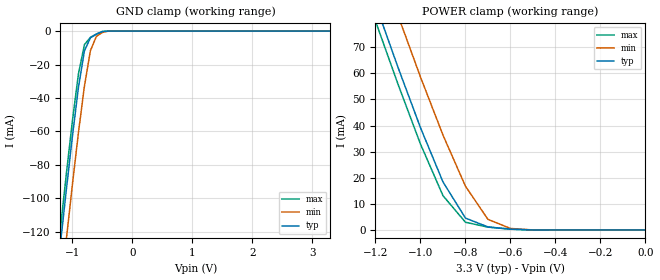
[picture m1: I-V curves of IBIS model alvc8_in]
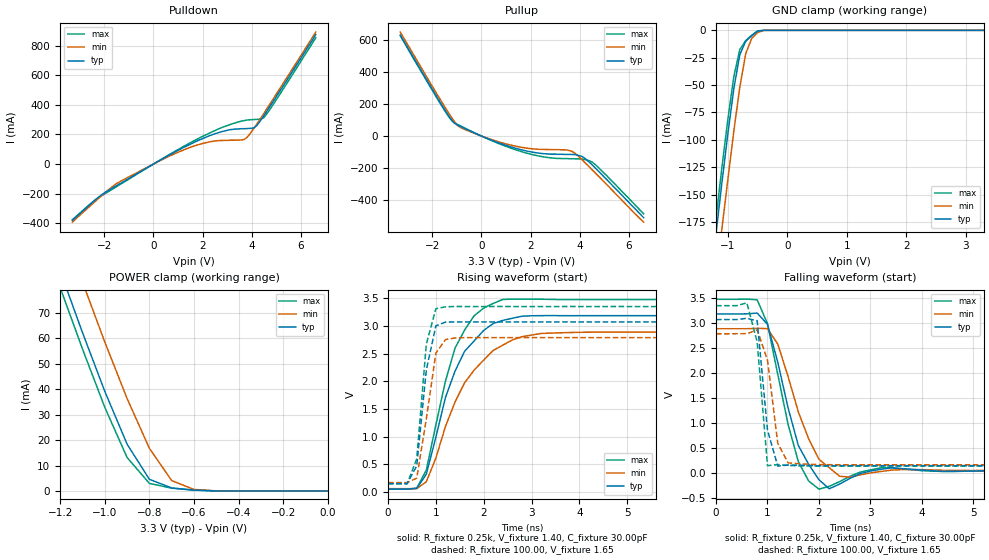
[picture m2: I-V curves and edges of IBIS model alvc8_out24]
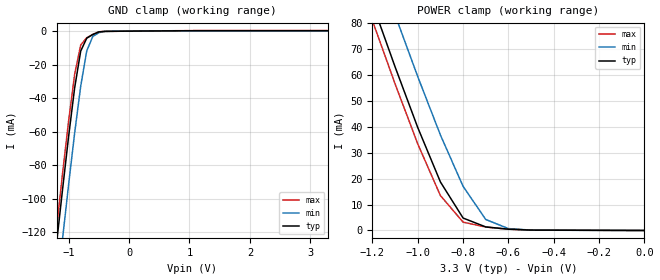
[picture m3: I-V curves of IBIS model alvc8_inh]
| IBIS file 16244ah.ibs created by s2ibis2 version 1.1
| North Carolina State University Electronics Research Laboratory  1995
[IBIS ver]   2.1
[File name]   16244ah.ibs
[File Rev]   1.0
[Date]   03/01/99 rtk rtk
[Source]   Integrated Device Technology, Inc.
[Notes]   1.Temperatures: typ=25C, min=100C, max=0C 2.RRmp rates based
   on 50 ohm load.
[Disclaimer] Integrated Device Technology, Inc. ("IDT") hereby grants the
   user of this IBIS model a non-exclusive, nontransferable
   license to use this IBIS model under the following terms. The
   user is granted this license only to use the IBIS model and is
   not granted rights to sell, copy (except as needed to run the
   IBIS model), rent, lease or sub-license the IBIS model in
   whole or in part, or in modified form to anyone. The User may
   modify the IBIS model to suit its specific applications, but
   rights to derivative works and such modifications shall belong
   to IDT. This IBIS model is provided on an AS IS" basis and IDT
   makes absolutely no warranty with respect to the information
   contained herein. IDT DISCLAIMS AND CUSTOMER WAIVES ALL
   WARRANTIES, EXPRESS AND IMPLIED, INCLUDING WARRANTIES OF
   MERCHANTABILITY AND FITNESS FOR A PARTICULAR PURPOSE. THE
   ENTIRE RISK AS TO QUALITY AND PERFORMANCE IS WITH THE USER
   ACCORDINGLY, IN NO EVENT SHALL IDT BE LIABLE FOR ANY DIRECT OR
   INDIRECT DAMAGES, WHETHER IN CONTRACT OR TORT, INCLUDING ANY
   LOST PROFITS OR OTHER INCIDENTAL, CONSEQUENTIAL, EXEMPLARY, OR
   PUNITIVE DAMAGES ARISING OUT OF THE USE OR APPLICATION OF THE
   IBIS model. Further, IDT reserves the right to make changes
   without notice to any product herein to improve reliability,
   function, or design. IDT does not convey any license under
   patent rights or any other intellectual property rights,
   including those of third parties. IDT is not obligated to
   provide maintenance or support for the licensed IBIS model.
[Copyright]   Copyright 1997, Integrated Device Technology, Inc. all rights
   reserved
|   Component ALVCH16244
[Component]   ALVCH16244
[Manufacturer]   Integrated Device Technology
[Package]
| PA48
| variable   typ   min   max
R_pkg   6.50m   5.00m   10.00m
L_pkg   3.20nH   2.50nH   4.40nH
C_pkg   0.27pF   0.01pF   0.98pF
| PV48   typ   min   max
|R_pkg   6.5m   5.00m   10.00m
|L_pkg   4.75nH   3.82nH   6.72nH
|C_pkg   0.24pF   0.01pF   1.55pF
[Pin]  signal_name   model_name   R_pin   L_pin   C_pin
1   1OEB   alvc8_in
2   1Y1   alvc8_out24
3   1Y2   alvc8_out24
4   GND   GND
5   1Y3   alvc8_out24
6   1Y4   alvc8_out24
7   VCC   POWER
8   2Y1   alvc8_out24
9   2Y2   alvc8_out24
10   GND   GND
11   2Y3   alvc8_out24
12   2Y4   alvc8_out24
13   3Y1   alvc8_out24
14   3Y2   alvc8_out24
15   GND   GND
16   3Y3   alvc8_out24
17   3Y4   alvc8_out24
18   VCC   POWER
19   4Y1   alvc8_out24
20   4Y2   alvc8_out24
21   GND   GND
22   4Y3   alvc8_out24
23   4Y4   alvc8_out24
24   4OEB   alvc8_in
25   3OEB   alvc8_in
26   4A4   alvc8_inh
27   4A3   alvc8_inh
28   GND   GND
29   4A2   alvc8_inh
30   4A1   alvc8_inh
31   VCC   POWER
32   3A4   alvc8_inh
33   3A3   alvc8_inh
34   GND   GND
35   3A2   alvc8_inh
36   3A1   alvc8_inh
37   2A4   alvc8_inh
38   2A3   alvc8_inh
39   GND   GND
40   2A2   alvc8_inh
41   2A1   alvc8_inh
42   VCC   POWER
43   1A4   alvc8_inh
44   1A3   alvc8_inh
45   GND   GND
46   1A2   alvc8_inh
47   1A1   alvc8_inh
48   2OEB   alvc8_in
| Models and submodels in the file (3): alvc8_in (Input), alvc8_out24 (3-state), alvc8_inh (Input)
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| in   in   dummy_model
| oe   oe   dummy_model
|   Model alvc8_in
[Model]   alvc8_in
Model_type   Input
Vinl =  0.800V
Vinh =  2.000V
C_comp   3.00pF   NA   NA
[Temperature Range]   25.00   100.00   0.000
[Voltage Range]   3.30V   3.00V   3.60V
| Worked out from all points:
|   GND clamp passes 1 mA (typ) near -0.54 V on its own axis
|   POWER clamp passes 1 mA (typ) near -0.68 V on its own axis
[GND_clamp]
| voltage   I(typ)   I(min)   I(max)
-3.3V     -860mA     -887mA     -851mA
-1.3V     -161mA     -190mA     -151mA
-1.2V     -127mA     -157mA     -118mA
-1.1V     -94.41mA   -124mA     -84.85mA
-1V       -62.78mA   -91.54mA   -53.52mA
-900mV    -33.71mA   -60.78mA   -25.6mA
-800mV    -11.74mA   -32.83mA   -8.09mA
-700mV    -4.033mA   -11.65mA   -3.7mA
-600mV    -1.899mA   -3.108mA   -1.699mA
-500mV    -308uA     -810uA     -172uA
-400mV    -3.848nA   -9.872uA   -399pA
3.3V      39.6pA     19.33nA    26.4pA
[POWER_clamp]
| voltage   I(typ)   I(min)   I(max)
-3.3V     630mA      648mA      624mA
-1.2V     86.56mA    106mA      80.02mA
-1.1V     62.33mA    82.22mA    55.88mA
-1V       39.2mA     58.61mA    32.91mA
-900mV    18.4mA     36.35mA    13.15mA
-800mV    4.556mA    16.76mA    2.954mA
-700mV    1.164mA    4.056mA    1.087mA
-600mV    320uA      578uA      299uA
-500mV    40.08nA    12.23uA    3.465nA
0V        39.6pA     59.11pA    43.2pA
|   Model alvc8_out24
[Model]   alvc8_out24
Model_type   3-state
Polarity   Non-Inverting
Enable   Active-High
Vmeas =  1.500V
C_comp   3.00pF   NA   NA
[Temperature Range]   25.00   100.00   0.000
[Voltage Range]   3.30V   3.00V   3.60V
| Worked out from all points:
|   slope of the pulldown table from 0 to 0.495 V, typ, clamps not added: 10.5 ohm
|   slope of the pullup table from 0 to 0.495 V, typ, clamps not added: 16.1 ohm
|   GND clamp passes 1 mA (typ) near -0.50 V on its own axis
|   POWER clamp passes 1 mA (typ) near -0.68 V on its own axis
|   rising waveform, R_fixture 0.25k, V_fixture 1.40, C_fixture 30.00pF: 20-80 % time 712ps typ, 930ps min, 636ps max; typ from 0.056 V to 3.19 V
|   rising waveform, R_fixture 100.00, V_fixture 1.65: 20-80 % time 241ps typ, 276ps min, 194ps max; typ from 0.155 V to 3.08 V
|   falling waveform, R_fixture 0.25k, V_fixture 1.40, C_fixture 30.00pF: 20-80 % time 456ps typ, 551ps min, 426ps max; typ from 3.19 V to 0.056 V
|   falling waveform, R_fixture 100.00, V_fixture 1.65: 20-80 % time 185ps typ, 189ps min, 171ps max; typ from 3.08 V to 0.155 V
[Pulldown]
| voltage   I(typ)   I(min)   I(max)
-3.3V     -381mA     -393mA     -377mA
-2.2V     -219mA     -227mA     -224mA
-1.5V     -146mA     -132mA     -153mA
500mV     47.5mA     41.7mA     49.9mA
1.4V      126mA      107mA      135mA
2.3V      193mA      151mA      211mA
3.1V      232mA      161mA      266mA
3.7V      239mA      167mA      294mA
4.1V      246mA      246mA      301mA
4.5V      329mA      345mA      316mA
5.1V      483mA      500mA      461mA
6.6V      875mA      892mA      853mA
[Pullup]
| voltage   I(typ)   I(min)   I(max)
-3.3V     630mA      649mA      628mA
-1.4V     142mA      160mA      137mA
-1.1V     80.6mA     90.7mA     83.6mA
-900mV    63mA       57.7mA     67.6mA
400mV     -25.1mA    -21.5mA    -27.4mA
1.6V      -85mA      -69.5mA    -95.9mA
2.6V      -111mA     -84mA      -132mA
3.4V      -115mA     -86.1mA    -141mA
3.7V      -115mA     -97.1mA    -142mA
4.1V      -128mA     -149mA     -144mA
4.5V      -179mA     -210mA     -162mA
6.6V      -510mA     -538mA     -486mA
[GND_clamp]
| voltage   I(typ)   I(min)   I(max)
-3.3V     -1.227A    -1.266A    -1.214A
-1.3V     -233mA     -276mA     -219mA
-1.2V     -186mA     -228mA     -172mA
-1.1V     -139mA     -181mA     -125mA
-1V       -94.27mA   -136mA     -81.1mA
-900mV    -53.23mA   -91.93mA   -42.09mA
-800mV    -22.31mA   -52.04mA   -17.61mA
-700mV    -9.958mA   -21.29mA   -9.325mA
-600mV    -4.943mA   -7.436mA   -4.424mA
-500mV    -830uA     -2.115mA   -472uA
-400mV    -8.73nA    -25.66uA   -695pA
3.3V      92.41pA    19.42nA    79.2pA
[POWER_clamp]
| voltage   I(typ)   I(min)   I(max)
-3.3V     630mA      648mA      624mA
-1.2V     86.56mA    106mA      80.02mA
-1.1V     62.33mA    82.22mA    55.88mA
-1V       39.2mA     58.61mA    32.91mA
-900mV    18.4mA     36.35mA    13.15mA
-800mV    4.556mA    16.76mA    2.954mA
-700mV    1.164mA    4.056mA    1.087mA
-600mV    320uA      578uA      299uA
-500mV    40.14nA    12.23uA    3.53nA
0V        92.41pA    138pA      101pA
[Ramp]
| variable   typ   min   max
dV/dt_r   1.48/0.31n   1.29/0.30n   1.66/0.22n
dV/dt_f   1.63/0.28n   1.45/0.31n   1.80/0.19n
R_load = 50.00
[Rising Waveform]
R_fixture = 0.25k
V_fixture = 1.40
C_fixture = 30.00pF
R_dut = 7.00m
L_dut = 3.30nH
C_dut = 0.29pF
| time   V(typ)   V(min)   V(max)
0s        55.61mV    62.15mV    53.22mV
600ps     67.1mV     63.76mV    71.36mV
800ps     323mV      188mV      399mV
1.2ns     1.71V      1.187V     2.006V
1.4ns     2.186V     1.627V     2.602V
1.8ns     2.733V     2.205V     3.187V
2.4ns     3.104V     2.656V     3.482V
2.8ns     3.179V     2.809V     3.489V
4ns       3.189V     2.888V     3.48V
19.8ns    3.189V     2.893V     3.481V
[Rising Waveform]
R_fixture = 100.00
V_fixture = 1.65
R_dut = 7.00m
L_dut = 3.30nH
C_dut = 0.29pF
| time   V(typ)   V(min)   V(max)
0s        155mV      173mV      149mV
400ps     155mV      173mV      149mV
600ps     476mV      252mV      604mV
800ps     2.207V     1.324V     2.674V
1ns       3.005V     2.511V     3.315V
1.2ns     3.072V     2.757V     3.349V
1.4ns     3.076V     2.786V     3.355V
1.6ns     3.076V     2.793V     3.354V
19.8ns    3.076V     2.792V     3.354V
[Falling Waveform]
R_fixture = 0.25k
V_fixture = 1.40
C_fixture = 30.00pF
R_dut = 7.00m
L_dut = 3.30nH
C_dut = 0.29pF
| time   V(typ)   V(min)   V(max)
0s        3.189V     2.893V     3.481V
800ps     3.206V     2.901V     3.471V
1ns       2.981V     2.895V     2.993V
1.2ns     2.223V     2.586V     1.98V
1.6ns     557mV      1.227V     234mV
2ns       -126mV     283mV      -314mV
2.2ns     -306mV     114mV      -257mV
2.4ns     -213mV     -54.48mV   -163mV
3.2ns     82.67mV    38.85mV    114mV
19.8ns    55.61mV    62.15mV    53.23mV
[Falling Waveform]
R_fixture = 100.00
V_fixture = 1.65
R_dut = 7.00m
L_dut = 3.30nH
C_dut = 0.29pF
| time   V(typ)   V(min)   V(max)
0s        3.076V     2.792V     3.354V
400ps     3.076V     2.793V     3.354V
600ps     3.101V     2.794V     3.411V
800ps     3.052V     2.869V     2.626V
1ns       869mV      2.268V     155mV
1.2ns     147mV      602mV      178mV
1.4ns     168mV      211mV      161mV
2ns       153mV      177mV      149mV
2.8ns     155mV      173mV      149mV
19.8ns    155mV      173mV      149mV
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|   Model alvc8_inh
[Model]   alvc8_inh
Model_type   Input
Vinl =  0.800V
Vinh =  2.000V
C_comp   3.00pF   NA   NA
[Temperature Range]   25.00   100.00   0.000
[Voltage Range]   3.30V   3.00V   3.60V
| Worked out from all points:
|   GND clamp passes 1 mA (typ) near -0.53 V on its own axis
|   POWER clamp passes 1 mA (typ) near -0.66 V on its own axis
[GND_clamp]
| voltage   I(typ)   I(min)   I(max)
-3.3V     -860mA     -888mA     -852mA
-1.3V     -161mA     -190mA     -151mA
-1.2V     -127mA     -157mA     -118mA
-1.1V     -94.51mA   -124mA     -84.99mA
-1V       -62.91mA   -91.62mA   -53.71mA
-900mV    -33.88mA   -60.87mA   -25.82mA
-800mV    -11.92mA   -32.93mA   -8.306mA
-700mV    -4.211mA   -11.77mA   -3.908mA
-600mV    -2.051mA   -3.213mA   -1.882mA
-500mV    -472uA     -914uA     -379uA
-400mV    -144uA     -112uA     -169uA
3.3V      264uA      163uA      349uA
[POWER_clamp]
| voltage   I(typ)   I(min)   I(max)
-3.3V     638mA      656mA      632mA
-1.2V     87.67mA    108mA      81.05mA
-1.1V     63.19mA    83.28mA    56.62mA
-1V       39.75mA    59.43mA    33.41mA
-900mV    18.73mA    36.86mA    13.47mA
-800mV    4.8mA      17.05mA    3.222mA
-700mV    1.374mA    4.243mA    1.32mA
-600mV    498uA      728uA      497uA
-500mV    146uA      134uA      162uA
0V        45.19pA    64.49pA    49.16pA
